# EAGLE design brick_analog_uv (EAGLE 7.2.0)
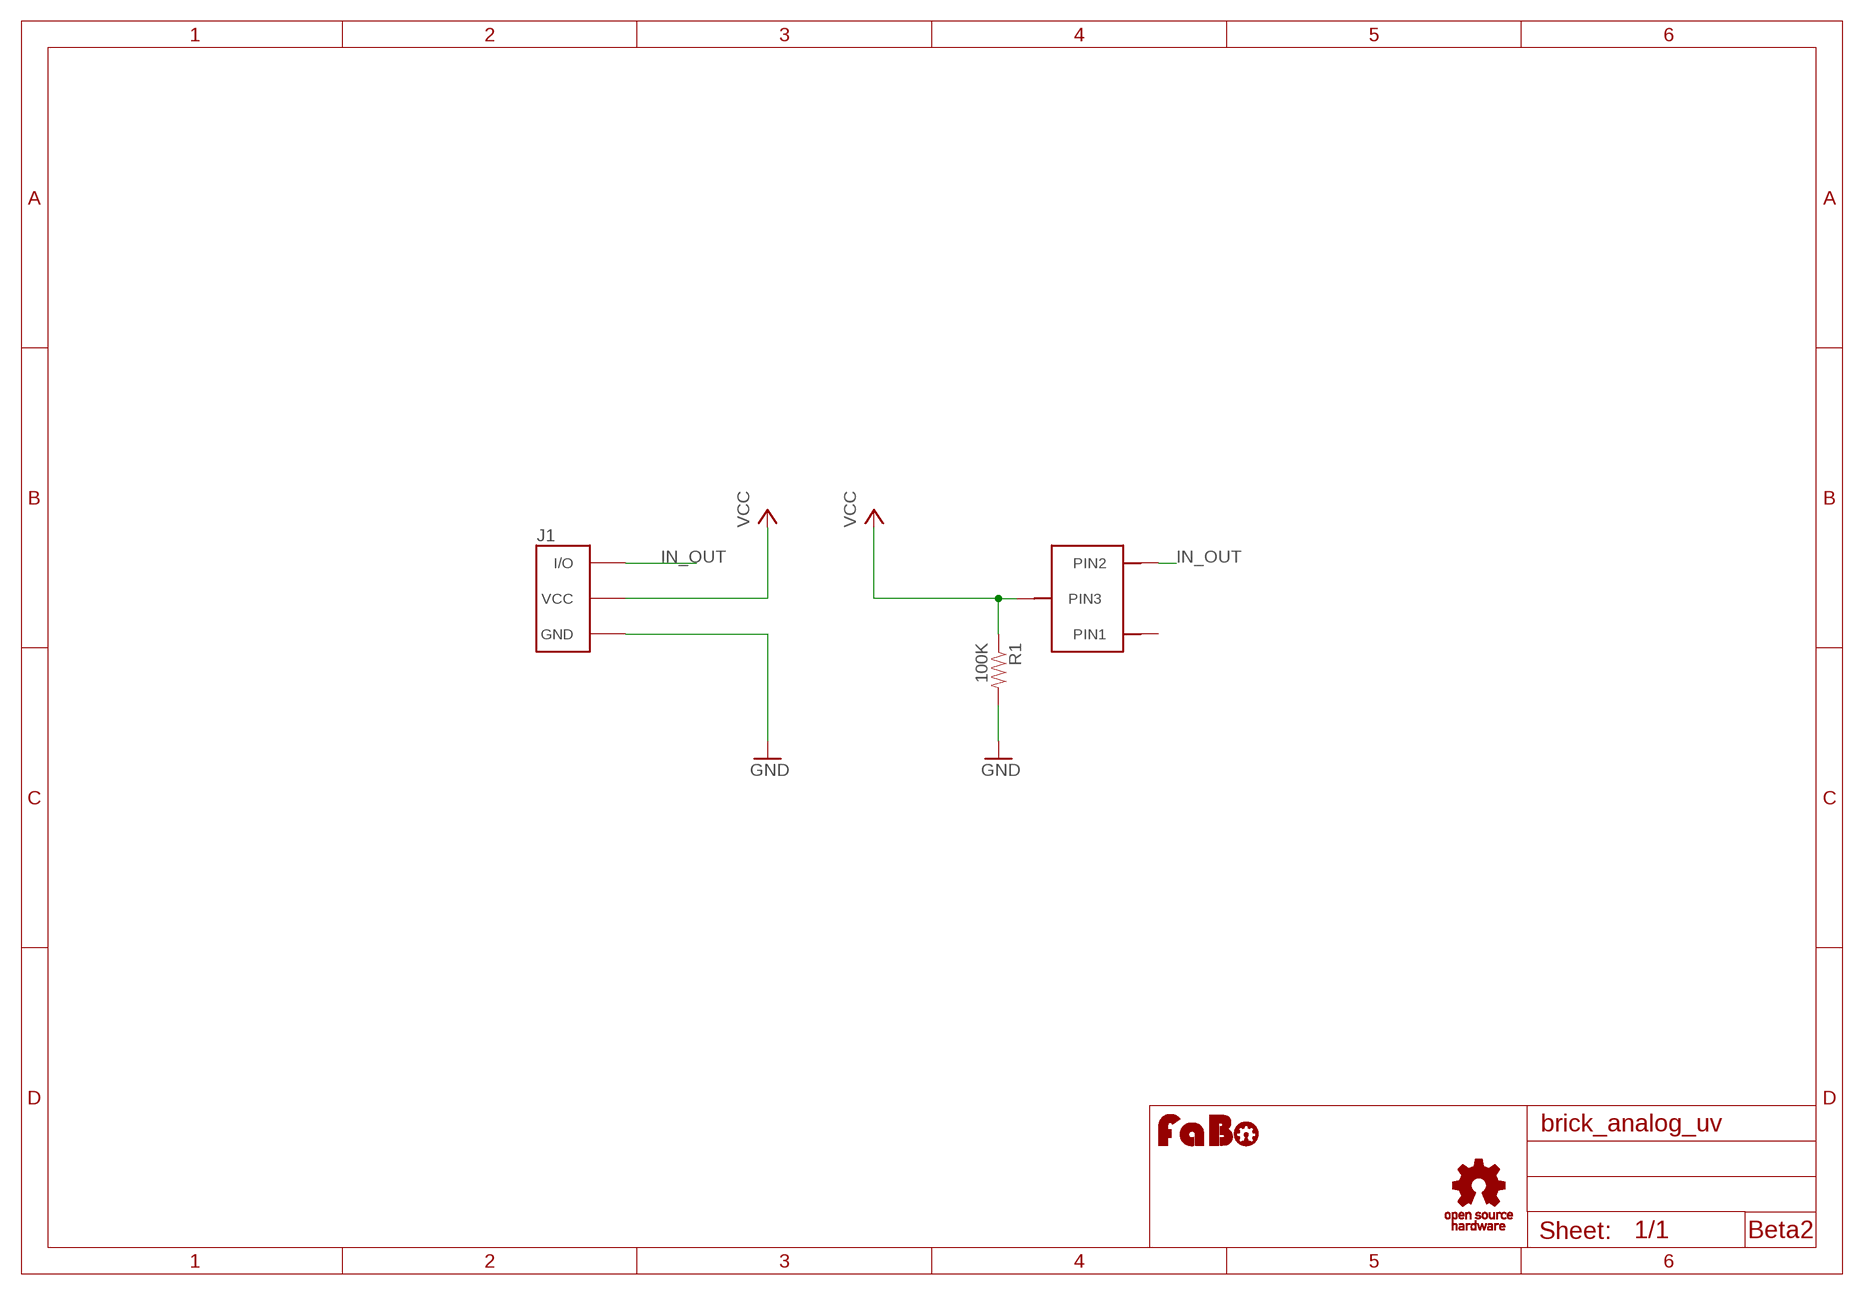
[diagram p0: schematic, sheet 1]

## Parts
J1  BRICK_3PIN  [BRICK_3PIN]
R1  100K  RESISTOR0603-RES  [0603-RES]
U1  HAMAMATSU-GAASP-G6262  [GAASP-G6262]
U$3  LOGO_OSHW_T-M  [LOGO_OSHW_T_M]
U$4  LOGO_FABO-M  [LOGO_FABO_M]

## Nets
GND: J1.GND R1.2
IN_OUT: J1.IN/OUT(I/O) U1.2(PIN2)
VCC: J1.VCC R1.1 U1.3(PIN3)
Unconnected: U1.1(PIN1)

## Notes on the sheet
- Beta2

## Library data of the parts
J1 = gclue:BRICK_3PIN: FaBo Brick 3pin
R1 = SparkFun:RESISTOR: Resistor
U1 = GClueSensor:HAMAMATSU-GAASP-G6262: GaAsP G6262
U$3 = gclue:LOGO_OSHW_T
U$4 = FaBo:LOGO_FABO

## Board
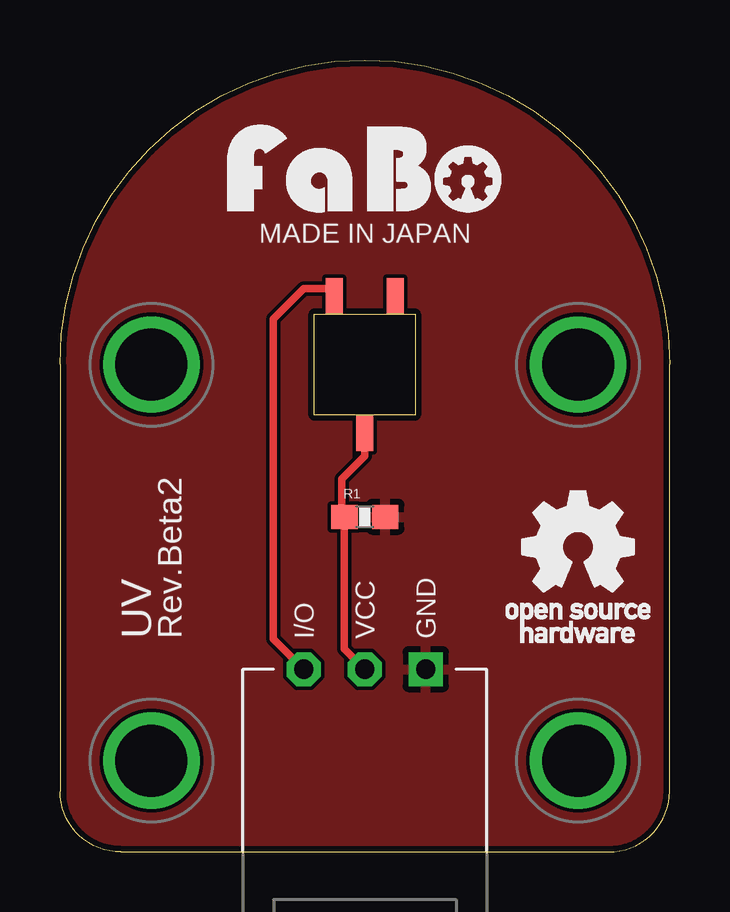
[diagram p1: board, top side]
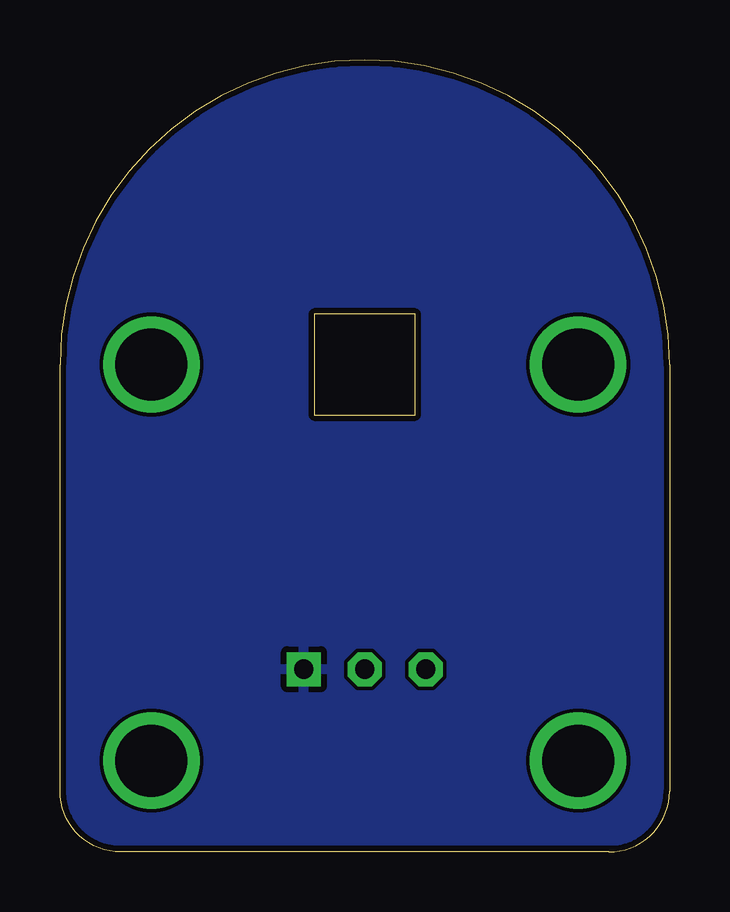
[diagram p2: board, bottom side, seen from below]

Size 25.4 x 33.02 mm. Coordinates in mm from the lower left corner, seen from the top.
Copper layers (1*16): Top 0.035mm / dielectric 1.5mm / Bottom 0.035mm
Design rules "Elecrow_2-layer_eagle_rule": minimum track width 6mil, minimum drill 12mil, track to track 6mil, track to pad 6mil, pad to pad 6mil, via to via 6mil, smd to smd 0mil, copper to edge 10mil, drill to drill 10mil, minimum pad ring 10mil, minimum via ring 6mil, stop-mask expansion 2mil, vias tented up to drill 100mil, thermal gap 10mil

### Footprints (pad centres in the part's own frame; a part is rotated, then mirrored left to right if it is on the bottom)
BRICK_3PIN = drill 0.8 pad 1.422 square: GND 2.54,-8.89 | drill 0.8 pad 1.422 octagon: IN/OUT -2.54,-8.89; VCC 0,-8.89 | drill 3 pad 3.81: P$5 -8.89,3.81; P$6 8.89,3.81; P$7 -8.89,-12.7; P$8 8.89,-12.7
0603-RES = smd 1.1 x 1: 1 -0.85,0; 2 0.85,0
GAASP-G6262 = smd 0.7 x 1.5: 1 -1.27,-2.85; 2 1.27,-2.85; 3 0,2.85

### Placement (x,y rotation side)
J1  12.7,16.51 0 top
R1  12.7,13.97 0 top
U1  12.7,20.32 180 top
U$3  21.59,12.7 0 top
U$4  12.7,26.67 0 top

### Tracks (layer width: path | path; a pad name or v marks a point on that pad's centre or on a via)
GND
  pour Bottom: -1.27,-1.27 26.67,-1.27 26.67,34.29 -1.27,34.29
  pour Top: -1.27,-1.27 26.67,-1.27 26.67,34.29 -1.27,34.29
IN_OUT
  Top 0.305: U1.2 11.43,23.5 10.16,23.5 8.89,22.23 8.89,8.89 J1.IN/OUT
VCC
  Top 0.305: J1.VCC 11.85,8.47 R1.1 11.75,14.29 11.75,15.56 12.7,16.51 U1.3

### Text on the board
tPlace: MADE IN JAPAN | UV | Rev.Beta2

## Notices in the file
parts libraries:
SparkFun: Licensing: CC v3.0 Share-Alike You are welcome to use this library for commercial purposes.
